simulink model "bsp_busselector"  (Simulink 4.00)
settings: Solver=ode45  SolverMode=SingleTasking  StartTime=0.0  StopTime=10.0  FixedStep=0.01  RelTol=1e-3

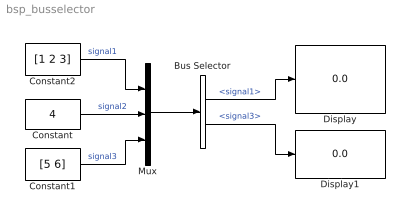
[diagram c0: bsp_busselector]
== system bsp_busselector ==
  Bus Selector : BusSelector  OutputSignals=signal1,signal3  MuxedOutput=off
  Constant : Constant  Value=4
  Constant1 : Constant  Value=[5 6]
  Constant2 : Constant  Value=[1 2 3]
  Display : Display
  Display1 : Display
  Mux : Mux  Inputs=3
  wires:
  Constant2/1 -> Mux/1  "signal1"
  Constant/1 -> Mux/2  "signal2"
  Constant1/1 -> Mux/3  "signal3"
  Mux/1 -> Bus Selector/1
  Bus Selector/1 -> Display/1  "<signal1>"
  Bus Selector/2 -> Display1/1  "<signal3>"
